PROGRAM EAP
VAR
	iEncode AT %I*	:UDINT;
	
	iEncode_Slaver AT %Q*	:UDINT;
	iCount AT %Q*	:UDINT;
	bWatchdog AT %Q*	:BOOL;
	bEnable AT %Q*	:BOOL;
	bReset AT %Q*	:BOOL;
	fbTON1: TON;
END_VAR

iCount:=iCount+1;	//用于测试通信延迟时间

//Master的心跳信号
fbTON1(IN:=NOT fbTON1.Q , PT:=T#50MS , Q=> , ET=> );
IF fbTON1.Q THEN
	bWatchdog:=NOT bWatchdog;
END_IF

iEncode_Slaver:=iEncode; //编码器信号送给从站

END_PROGRAM
